(* Logix 5000 DataType export R203_Seneca_OutData; software revision 35.00 *)

TYPE R203_Seneca_OutData :   // User Define Data Out Type for Seneca R203-E Advanced Power Meter Device
STRUCT
   DOUT1 : BOOL;   // Digital Output1
   DOUT2 : BOOL;   // Digital Output2
   NOT_USED_2 : BOOL;   // Not used
   NOT_USED_3 : BOOL;   // Not used
   NOT_USED_4 : BOOL;   // Not used
   NOT_USED_5 : BOOL;   // Not used
   NOT_USED_6 : BOOL;   // Not used
   NOT_USED_7 : BOOL;   // Not used
   UNUSED_BYTE1 : SINT;   // Not Used
   UNUSED_BYTE2 : SINT;   // Not Used
   UNUSED_BYTE3 : SINT;   // Not Used
   ANALOG_OUTPUT_mV_uA : REAL;   // Analog Output value [mV] or [uA]
   CMD_AUX : UDINT;   // Command AUX
   CMD : UDINT;   // Command Register
END_STRUCT
END_TYPE
